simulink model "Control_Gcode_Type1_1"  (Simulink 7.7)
settings: Solver=FixedStepDiscrete  SolverMode=SingleTasking  StartTime=0  StopTime=inf  FixedStep=dt  RelTol=1e-3  SampleTimeConstraint=Specified
InitFcn:
  | % Sampling Times %
  | dt0=0.001; dt1=0.01; samples=10;
undefined symbols (not defined in the file or in its folder): DiscIntNeverNeededParam, Volts
libraries: simulink_extras x4, speedgoatlib_IO311 x3, xpclib x3, speedgoatlib x2, simulink x2

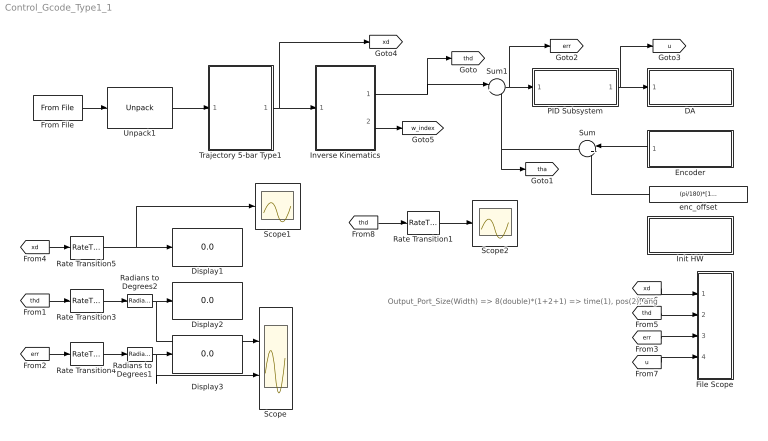
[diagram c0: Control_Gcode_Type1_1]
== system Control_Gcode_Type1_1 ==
  note: Output_Port_Size(Width) => 8(double)*(1+2+1) => time(1), pos(2), ang
  DA : Subsystem  TreatAsAtomicUnit=on
  Display1 : Display
  Display2 : Display
  Display3 : Display
  Encoder : Subsystem  TreatAsAtomicUnit=on
  File Scope : Subsystem
  From File : xpclib/Misc./From File  filename='five1.dat'  dataSize=32  bufSize=4000  readSize=1024  EOFOption=Hold last output  sampTime=dt0
  Init HW : Subsystem  TreatAsAtomicUnit=on
  Inverse Kinematics : Stateflow chart  TreatAsAtomicUnit=on
  PID Subsystem : Subsystem  TreatAsAtomicUnit=on
  Radians to Degrees1 : simulink_extras/Transformations/Radians to Degrees  SystemSampleTime=-1
  Radians to Degrees2 : simulink_extras/Transformations/Radians to Degrees  SystemSampleTime=-1
  Rate Transition{1,3..5} (4 alike) : RateTransition  OutPortSampleTime=dt1
  Scope : Scope  NumInputPorts=2
  Scope1 : Scope
  Scope2 : Scope
  Sum : Sum  Inputs=|++
  Sum1 : Sum  Inputs=|+-
  Trajectory 5-bar Type1 : Stateflow chart  TreatAsAtomicUnit=on
  Unpack1 : xpclib/UDP/Unpack  dimensions={[4]}  datatypes={'double'}  byteAlign=1
  enc_offset : Constant  Value=(pi/180)*[118.81,61.19]'
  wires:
  [thd] -> Rate Transition3/1
  [err] -> Rate Transition4/1
  [xd] -> Rate Transition5/1
  Rate Transition5/1 -> Display1/1, Scope1/1
  Rate Transition3/1 -> Radians to Degrees2/1
  Rate Transition4/1 -> Radians to Degrees1/1
  Radians to Degrees2/1 -> Display2/1, Scope/1
  Radians to Degrees1/1 -> Display3/1, Scope/2
  [xd] -> File Scope/1(xd)
  [thd] -> File Scope/2(thd)
  [err] -> File Scope/3(err)
  [u] -> File Scope/4(u)
  From File/1 -> Unpack1/1
  Unpack1/1 -> Trajectory 5-bar Type1/1(traj)
  Sum1/1 -> PID Subsystem/1(In1), [err]
  PID Subsystem/1(Out1) -> [u], DA/1(In1)
  Encoder/1(Out1) -> Sum/1
  enc_offset/1 -> Sum/2
  Sum/1 -> Sum1/2, [tha]
  Trajectory 5-bar Type1/1(xd) -> [xd], Inverse Kinematics/1(xd)
  Inverse Kinematics/1(thd) -> Sum1/1, [thd]
  Inverse Kinematics/2(w_index) -> [w_index]
  [thd] -> Rate Transition1/1
  Rate Transition1/1 -> Scope2/1

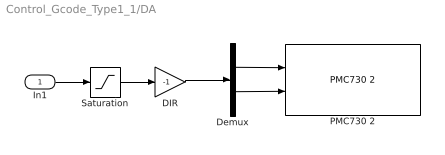
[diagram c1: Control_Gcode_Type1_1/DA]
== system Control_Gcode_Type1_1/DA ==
  In1 : Inport
  DIR : Gain  Gain=-1
  Demux : Demux  Outputs=2
  PMC730 2 : speedgoatlib/IO101/PMC730 2  id=1  channel=[1,2]  reset=[1,1]  initValue=[0,0]  ts=dt0  pciSlot=-1
  Saturation : Saturate  UpperLimit=10  LowerLimit=-10
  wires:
  In1/1 -> Saturation/1
  Saturation/1 -> DIR/1
  DIR/1 -> Demux/1
  Demux/1 -> PMC730 2/1
  Demux/2 -> PMC730 2/2

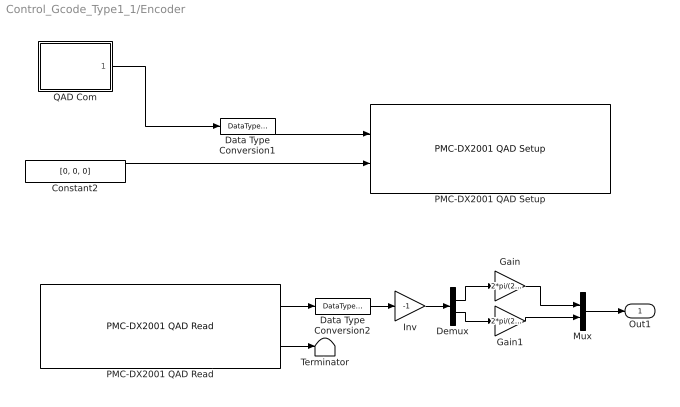
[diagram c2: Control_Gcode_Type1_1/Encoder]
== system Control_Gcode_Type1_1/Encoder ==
  Constant2 : Constant  Value=[0, 0, 0]  OutDataTypeStr=Inherit: Inherit via back propagation
  Data Type Conversion1 : DataTypeConversion  OutDataTypeStr=uint8
  Data Type Conversion2 : DataTypeConversion  OutDataTypeStr=double
  Demux : Demux  Outputs=2
  Gain : Gain  Gain=2*pi/(23*2000)
  Gain1 : Gain  Gain=2*pi/(23*2000)
  Inv : Gain  Gain=-1
  Mux : Mux  Inputs=2
  PMC-DX2001 QAD Read : speedgoatlib_IO311/PMC-DX2001 QAD Read  id=1  chan=[1, 2]  pciSlot=-1  ts=dt0
  PMC-DX2001 QAD Setup : speedgoatlib_IO311/PMC-DX2001 QAD Setup  id=1  chan=Channel 3 setup  steps1=2000  steps2=2000  steps3=2000  quadrature1=4x  quadrature2=4x  quadrature3=4x  index1=Ignore index input  index2=Ignore index input  index3=Ignore index input  special1=Disabled (cycling counter)  special2=Disabled (cycling counter)  special3=Disabled (cycling counter)  debounce=0  pciSlot=-1  ts=dt0
  QAD Com : Stateflow chart  TreatAsAtomicUnit=on
  Terminator : Terminator
  Out1 : Outport
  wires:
  Constant2/1 -> PMC-DX2001 QAD Setup/2
  PMC-DX2001 QAD Read/2 -> Terminator/1
  PMC-DX2001 QAD Read/1 -> Data Type Conversion2/1
  QAD Com/1(y) -> Data Type Conversion1/1
  Data Type Conversion1/1 -> PMC-DX2001 QAD Setup/1
  Data Type Conversion2/1 -> Inv/1
  Mux/1 -> Out1/1
  Demux/1 -> Gain/1
  Gain/1 -> Mux/1
  Demux/2 -> Gain1/1
  Gain1/1 -> Mux/2
  Inv/1 -> Demux/1

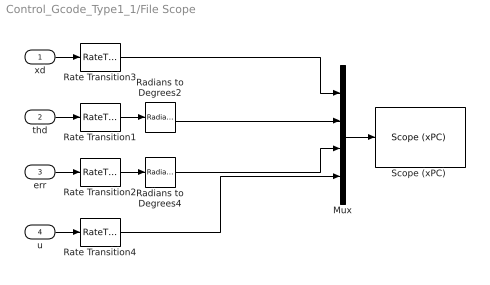
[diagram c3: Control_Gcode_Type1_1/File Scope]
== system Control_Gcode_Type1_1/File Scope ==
  xd : Inport
  thd : Inport  Port=2
  err : Inport  Port=3
  u : Inport  Port=4
  Mux : Mux
  Radians to Degrees2 : simulink_extras/Transformations/Radians to Degrees  SystemSampleTime=-1
  Radians to Degrees4 : simulink_extras/Transformations/Radians to Degrees  SystemSampleTime=-1
  Rate Transition{1..4} (4 alike) : RateTransition  OutPortSampleTime=dt1
  "Scope (xPC) " : xpclib/Misc./Scope (xPC)   SystemSampleTime=-1  scopeno=2  scopetype=File  autostart=on  viewmode=Graphical redraw  formatstr='%15.6f'  grid=on  ylimits=[0,0]  nosamples=100  noprepostsamples=0  interleave=1  triggermode=FreeRun  triggersignal=1  triggerlevel=0.0  triggerslope=Either  triggerscope=1  triggersample=0  filename=step3.dat  mode=Lazy  writesize=512  autorestart=on  dynamicfilemode=off  maxwritefilesize=512*1024^2
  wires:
  Radians to Degrees2/1 -> Mux/2
  Radians to Degrees4/1 -> Mux/3
  Rate Transition1/1 -> Radians to Degrees2/1
  Rate Transition2/1 -> Radians to Degrees4/1
  thd/1 -> Rate Transition1/1
  err/1 -> Rate Transition2/1
  Rate Transition3/1 -> Mux/1
  xd/1 -> Rate Transition3/1
  u/1 -> Rate Transition4/1
  Mux/1 -> "Scope (xPC) "/1
  Rate Transition4/1 -> Mux/4

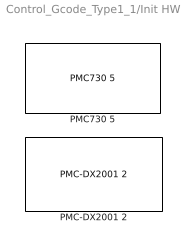
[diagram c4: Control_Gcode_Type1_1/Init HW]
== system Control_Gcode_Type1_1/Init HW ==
  PMC-DX2001 2 : speedgoatlib_IO311/PMC-DX2001 2  id=1  fpga1=IO311_3PWM_3CAP_3QAD_INT.fpga  fpga2=PWM_Triangle_DX501.fpga  fpga3=PWM_Triangle_DX501.fpga  fpga4=PWM_Triangle_DX501.fpga  fpga5=PWM_Triangle_DX501.fpga  fpga6=PWM_Triangle_DX501.fpga  fpga7=PWM_Triangle_DX501.fpga  fpga8=PWM_Triangle_DX501.fpga  fpga9=PWM_Triangle_DX501.fpga  fpga10=PWM_Triangle_DX501.fpga  group=Module setup  pciSlot=-1  lowerDirection=[ones(1,5), zeros(1, 7), ones(1, 1), ones(1, 3)]  lowerReset=[1]  lowerValue=[0]  upperDirection=[ones(1, 8), zeros(1, 8)]  upperReset=[1]  upperValue=[0]
  PMC730 5 : speedgoatlib/IO101/PMC730 5  id=1  group=Analog output setup  pciSlot=-1  adStartChannel=1  adNumChannel=1  adCoupling=Single-ended  adRange=-10 .. 10 Volts  adAcqMode=Standard  daChannel=[1,2]  daReset=[1,1]  daInitValue=[0,0]  diChannel=[1]  diDebounce=[0]  doChannel=[1]  doReset=[1]  doInitValue=[0]

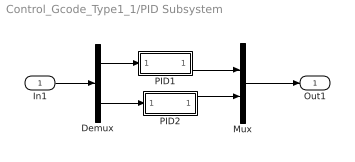
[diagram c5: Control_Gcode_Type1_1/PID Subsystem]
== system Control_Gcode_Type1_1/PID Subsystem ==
  In1 : Inport
  Demux : Demux  Outputs=2
  Mux : Mux  Inputs=2
  PID1 : Subsystem
  PID2 : Subsystem
  Out1 : Outport
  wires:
  In1/1 -> Demux/1
  Demux/1 -> PID1/1(In1)
  PID1/1(Out1) -> Mux/1
  Demux/2 -> PID2/1(In1)
  PID2/1(Out1) -> Mux/2
  Mux/1 -> Out1/1

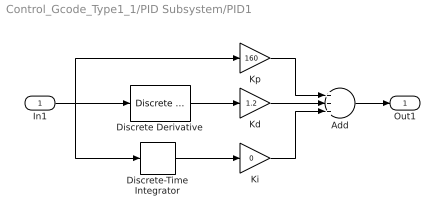
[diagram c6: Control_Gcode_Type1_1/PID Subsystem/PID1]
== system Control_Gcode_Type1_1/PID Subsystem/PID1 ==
  In1 : Inport
  Add : Sum  Inputs=+++
  Discrete Derivative : simulink/Discrete/Discrete Derivative  SystemSampleTime=-1  gainval=1.0  ICPrevScaledInput=0.0  OutMin=[]  OutMax=[]  OutDataType=fixdt(1, 16)  OutScaling=2^-10  DoSatur=off
  Discrete-Time Integrator : DiscreteIntegrator  SampleTime=dt0  ICPrevOutput=DiscIntNeverNeededParam  ICPrevScaledInput=DiscIntNeverNeededParam
  Kd : Gain  Gain=1.2
  Ki : Gain  Gain=0
  Kp : Gain  Gain=160
  Out1 : Outport
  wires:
  Discrete-Time Integrator/1 -> Ki/1
  Kp/1 -> Add/1
  Kd/1 -> Add/2
  Ki/1 -> Add/3
  Discrete Derivative/1 -> Kd/1
  Add/1 -> Out1/1
  In1/1 -> Kp/1, Discrete Derivative/1, Discrete-Time Integrator/1

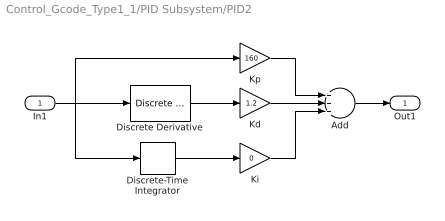
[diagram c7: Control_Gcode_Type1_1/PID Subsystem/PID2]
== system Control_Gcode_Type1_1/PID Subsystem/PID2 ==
  In1 : Inport
  Add : Sum  Inputs=+++
  Discrete Derivative : simulink/Discrete/Discrete Derivative  SystemSampleTime=-1  gainval=1.0  ICPrevScaledInput=0.0  OutMin=[]  OutMax=[]  OutDataType=fixdt(1, 16)  OutScaling=2^-10  DoSatur=off
  Discrete-Time Integrator : DiscreteIntegrator  SampleTime=dt0  ICPrevOutput=DiscIntNeverNeededParam  ICPrevScaledInput=DiscIntNeverNeededParam
  Kd : Gain  Gain=1.2
  Ki : Gain  Gain=0
  Kp : Gain  Gain=160
  Out1 : Outport
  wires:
  Discrete-Time Integrator/1 -> Ki/1
  Kp/1 -> Add/1
  Kd/1 -> Add/2
  Ki/1 -> Add/3
  Discrete Derivative/1 -> Kd/1
  Add/1 -> Out1/1
  In1/1 -> Kp/1, Discrete Derivative/1, Discrete-Time Integrator/1

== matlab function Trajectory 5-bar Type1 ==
function xd = fcn(traj)

%x0=[48.5600, 168.2722]';
x0=[60.8523, 154.6652]';
xd=x0+traj(2:3,1);

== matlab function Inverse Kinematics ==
function [thd,w_index]  = fcn(xd)

persistent index thd_p
persistent th3_p th4_p

% Initializing Variables %
if isempty(index), index=0; end
if isempty(thd_p), thd_p=(pi/180)*[118.81,61.19]'; end
if isempty(th3_p), th3_p=0; end
if isempty(th4_p), th4_p=0; end

% Kinematic Parameters %
L1=74;  % 54 --> 74
L2=100; L3=100; L4=100; L5=100; L6=28;

w_index=1;  % In workspace %

% (1) Left Side 2-DOF Arm %
px=xd(1,1); py=xd(2,1);
k1=(px^2+py^2-L2^2-(L3+L6)^2)/(2*L2*(L3+L6));
if abs(k1)<=1
    th3=-acos(k1);
else
    w_index=-1;
    th3=th3_p;
end

DEL1=L2^2+(L3+L6)^2+2*L2*(L3+L6)*cos(th3);
cth2=(px*(L2+(L3+L6)*cos(th3))+py*(L3+L6)*sin(th3))/DEL1;
sth2=(-px*(L3+L6)*sin(th3)+py*(L2+(L3+L6)*cos(th3)))/DEL1;
th2=atan2(sth2,cth2);

% (2) Right Side 2-DOF Arm %
cx=px-L6*cos(th2+th3)-L1; cy=py-L6*sin(th2+th3);
k2=(cx^2+cy^2-L5^2-L4^2)/(2*L5*L4);
if abs(k2)<=1
    th4=acos(k2);
else
    w_index=-2;
    th4=th4_p;
end

DEL2=L5^2+L4^2+2*L5*L4*cos(th4);
cth5=(cx*(L5+L4*cos(th4))+cy*L4*sin(th4))/DEL2;
sth5=(-cx*L4*sin(th4)+cy*(L5+L4*cos(th4)))/DEL2;
th5=atan2(sth5,cth5);

% Result %
if w_index==1
    thd=[th2, th5]';
else
    thd=thd_p;
end

% Save the current value %
thd_p=thd;
th3_p=th3; th4_p=th4;

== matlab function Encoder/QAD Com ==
function y = fcn()

persistent index

if isempty(index), index=0; end

if index==0
    y=[1,1,1];      %  Reset %
else
    y = [0,0,0];
end

index=index+1;
